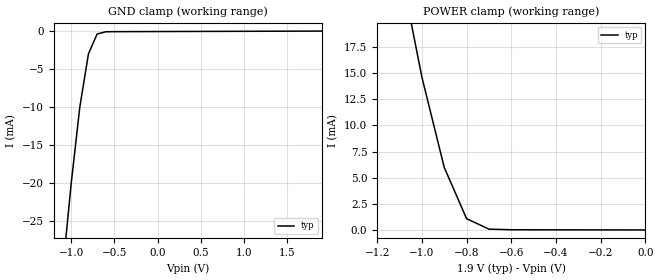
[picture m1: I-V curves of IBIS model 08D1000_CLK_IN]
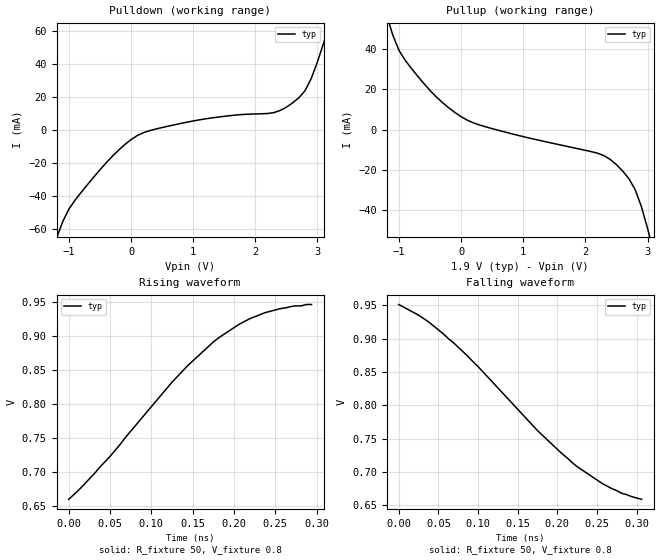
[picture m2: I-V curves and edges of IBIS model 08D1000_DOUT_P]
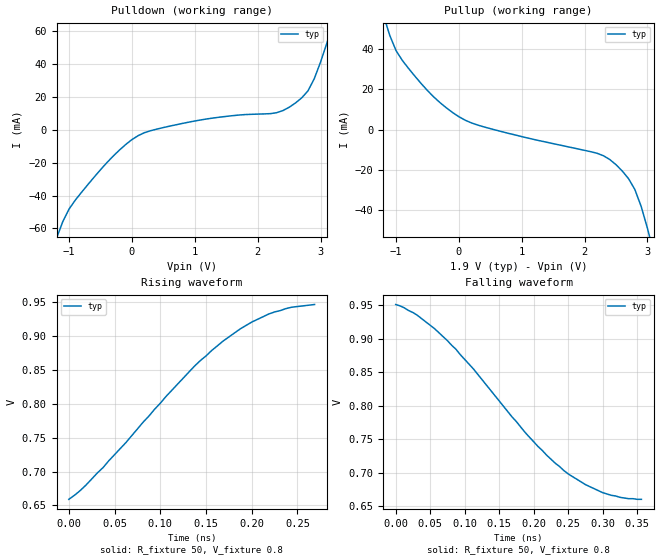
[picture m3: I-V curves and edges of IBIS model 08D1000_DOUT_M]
|   National Semiconductor Corporation
|   Data Conversion Products Group
|   IBIS Model of ADC08D1000
|   128 Pin Exposed Pad LQFP Package
[IBIS Ver]   3.2
[File name]   adc08d1000.ibs
[File Rev]   1.1
[Date]   08/11/06
[Source]   Bench Test to Ibis Conversion.
[Notes]   File created by Ian King
   Updated by Craig Klem  -  Fixed [Diff-pin] to allow
   LineSim simulations
[Disclaimer]
(C) Copyright National Semiconductor Corporation 2006
   All rights reserved
   National Semiconductor Corporation hereby grants
the user of this IBIS model a non-exclusive, nontransferable
license to use this IBIS model under the following terms.
Before using this IBIS model, the user should read this
license.  If the user does not accept these terms,  the
IBIS model should be returned to National within 30 days.
   The user is granted this license only to use the
IBIS model and is not granted rights to sell, load, rent,
lease or license the IBIS model in whole or in part, or in
modified form to anyone other than user. User may modify
the IBIS model to suit its specific applications but rights
to derivative works and such modifications shall belong to
National.
   This IBIS model is provided on an "AS IS" basis and
National makes absolutely no warranty with respect to the
information contained herein.NATIONAL DISCLAIMS AND CUSTOMER
WAIVES ALL WARRANTIES, EXPRESS OR IMPLIED, INCLUDING
WARRANTIES OF MERCHANTABILITY OR FITNESS FOR A PARTICULAR
PURPOSE. The entire risk as to quality and performance is
with the Customer. ACCORDINGLY, IN NO EVENT SHALL THE
COMPANY BE LIABLE FOR ANY DAMAGES, WHETHER IN CONTRACT OR
TORT,INCLUDING ANY LOST PROFITS OR OTHER INCIDENTAL,
CONSEQUENTIAL, EXEMPLARY, OR PUNITIVE DAMAGES ARISING OUT
OF THE USE OR APPLICATION OF THE IBIS model provided in
this package.Further, National reserves the right to make
changes without notice to any product herein to improve
reliability, function, or design. National does not convey
any license under patent rights or any other intellectual
property rights, including those of third parties.
   National is not obligated to provide maintenance or support
for the licensed IBIS model.
Contact National at ATTN:DCS APPLICATIONS/IBIS MODELS.
2900 Semiconductor Drive, M/S D3-739, Santa Clara, CA 95052-8090
[Copyright]   Copyright 2006, National Semiconductor, All Rights Reserved
[Component]   ADC08D1000
[Manufacturer]  National Semiconductor Corp
[Package]
|   typ   min   max
R_pkg   416.0m   397.0m   444.0m
L_pkg   8.66n   7.94n   10.10n
C_pkg   0.10p   0.09p   0.14p
[Pin]   signal_name   model_name   R_pin   L_pin   C_pin
1   GND   GND   426.0m   10.1n   0.14p
2   VA   POWER   431.0m   9.78n   0.12p
3   OUTV/SCLK   NC
4   OE/DDR/SDATA   NC
5   VA   POWER   444.0m   9.14n   0.10p
6   GND   GND   435.0m   8.93n   0.10p
7   VCMO   NC
8   VA   POWER   417.0m   8.52n   0.10p
9   GND   GND   408.0m   8.31n   0.10p
10   VINI-   NC   407.0m   8.23n   0.10p
11   VINI+   NC   403.0m   8.18n   0.10p
12   GND   GND   397.0m   7.94n   0.10p
13   VA   POWER   397.0m   8.04n   0.09p
14   FSR/ECE   NC
15   DCLK_RST   NC
16   VA   POWER   397.0m   7.99n   0.09p
17   VA   POWER   397.0m   7.99n   0.09p
18   CLK+   08D1000_CLK_IN   397.0m   7.99n   0.09p
19   CLK-   08D1000_CLK_IN   397.0m   7.99n   0.09p
20   VA   POWER   397.0m   8.04n   0.09p
21   GND   GND   397.0m   7.94n   0.10p
22   VINQ+   NC   403.0m   8.18n   0.10p
23   VINQ-   NC   407.0m   8.23n   0.10p
24   GND   GND   408.0m   8.31n   0.10p
25   VA   POWER   417.0m   8.52n   0.10p
26   PD   NC
27   GND   GND   435.0m   8.93n   0.10p
28   VA   POWER   444.0m   9.14n   0.10p
29   PDQ   NC
30   CAL   NC
31   VBG   NC
32   REXT   NC
33   VA   POWER   426.0m   10.1n   0.14p
34   TDIODE_P   NC
35   TDIODE_N   NC
36   DQD0+   08D1000_DOUT_P   444.0m   9.27n   0.10p
37   DQD0-   08D1000_DOUT_M   444.0m   9.14n   0.10p
38   DQD1+   08D1000_DOUT_P   435.0m   8.93n   0.10p
39   DQD1-   08D1000_DOUT_M   426.0m   8.73n   0.10p
40   VDR   POWER   417.0m   8.52n   0.10p
41   GND   GND   408.0m   8.31n   0.10p
42   DRGND   GND   407.0m   8.23n   0.10p
43   DQD2+   08D1000_DOUT_P   403.0m   8.18n   0.10p
44   DQD2-   08D1000_DOUT_M   397.0m   7.94n   0.10p
45   DQD3+   08D1000_DOUT_P   397.0m   8.04n   0.09p
46   DQD3-   08D1000_DOUT_M   397.0m   7.99n   0.09p
47   DQD4+   08D1000_DOUT_P   397.0m   7.99n   0.09p
48   DQD4-   08D1000_DOUT_M   397.0m   7.99n   0.09p
49   DQD5+   08D1000_DOUT_P   397.0m   7.99n   0.09p
50   DQD5-   08D1000_DOUT_M   397.0m   7.99n   0.09p
51   VDR   POWER   397.0m   7.99n   0.09p
52   NC   NC
53   DRGND   GND   397.0m   7.94n   0.10p
54   DQD6+   08D1000_DOUT_P   403.0m   8.18n   0.10p
55   DQD6-   08D1000_DOUT_M   407.0m   8.23n   0.10p
56   DQD7+   08D1000_DOUT_P   408.0m   8.31n   0.10p
57   DQD7-   08D1000_DOUT_M   417.0m   8.52n   0.10p
58   DQ0+   08D1000_DOUT_P   426.0m   8.73n   0.10p
59   DQ0-   08D1000_DOUT_M   435.0m   8.93n   0.10p
60   DQ1+   08D1000_DOUT_P   444.0m   9.14n   0.10p
61   DQ1-   08D1000_DOUT_M   444.0m   9.27n   0.10p
62   VDR   POWER   436.0m   9.78n   0.10p
63   NC   NC
64   DRGND   GND   426.0m   10.1n   0.14p
65   DQ2+   08D1000_DOUT_P   426.0m   10.1n   0.14p
66   DQ2-   08D1000_DOUT_M   431.0m   9.78n   0.12p
67   DQ3+   08D1000_DOUT_P   436.0m   9.42n   0.10p
68   DQ3-   08D1000_DOUT_M   444.0m   9.27n   0.10p
69   DQ4+   08D1000_DOUT_P   444.0m   9.14n   0.10p
70   DQ4-   08D1000_DOUT_M   435.0m   8.93n   0.10p
71   DQ5+   08D1000_DOUT_P   426.0m   8.73n   0.10p
72   DQ5-   08D1000_DOUT_M   417.0m   8.52n   0.10p
73   VDR   POWER   408.0m   8.31n   0.10p
74   DRGND   GND   407.0m   8.23n   0.10p
75   DQ6+   08D1000_DOUT_P   403.0m   8.18n   0.10p
76   DQ6-   08D1000_DOUT_M   397.0m   7.94n   0.10p
77   DQ7+   08D1000_DOUT_P   397.0m   7.99n   0.09p
78   DQ7-   08D1000_DOUT_M   397.0m   7.99n   0.09p
79   OR+   NC
80   OR-   NC
81   DCLK-   08D1000_DCLK_M   397.0m   7.99n   0.09p
82   DCLK+   08D1000_DCLK_P   397.0m   7.99n   0.09p
83   DI7-   08D1000_DOUT_M   397.0m   7.99n   0.09p
84   DI7+   08D1000_DOUT_P   397.0m   8.04n   0.09p
85   DI6-   08D1000_DOUT_M   397.0m   7.94n   0.10p
86   DI6+   08D1000_DOUT_P   403.0m   8.18n   0.10p
87   DRGND   GND   407.0m   8.23n   0.10p
88   VDR   POWER   408.0m   8.31n   0.10p
89   DI5-   08D1000_DOUT_M   417.0m   8.52n   0.10p
90   DI5+   08D1000_DOUT_P   426.0m   8.73n   0.10p
91   DI4-   08D1000_DOUT_M   435.0m   8.93n   0.10p
92   DI4+   08D1000_DOUT_P   444.0m   9.14n   0.10p
93   DI3-   08D1000_DOUT_M   444.0m   9.27n   0.10p
94   DI3+   08D1000_DOUT_P   436.0m   9.42n   0.10p
95   DI2-   08D1000_DOUT_M   431.0m   9.78n   0.12p
96   DI2+   08D1000_DOUT_P   426.0m   10.1n   0.14p
97   DRGND   GND   426.0m   10.1n   0.14p
98   NC   NC
99   VDR   POWER   436.0m   9.42n   0.10p
100   DI1-   08D1000_DOUT_M   444.0m   9.27n   0.10p
101   DI1+   08D1000_DOUT_P   444.0m   9.14n   0.10p
102   DI0-   08D1000_DOUT_M   435.0m   8.93n   0.10p
103   DI0+   08D1000_DOUT_P   426.0m   8.73n   0.10p
104   DID7-   08D1000_DOUT_M   417.0m   8.52n   0.10p
105   DID7+   08D1000_DOUT_P   408.0m   8.31n   0.10p
106   DID6-   08D1000_DOUT_M   407.0m   8.23n   0.10p
107   DID6+   08D1000_DOUT_P   403.0m   8.18n   0.10p
108   DRGND   GND   397.0m   7.94n   0.10p
109   NC   NC
110   VDR   POWER   397.0m   7.99n   0.09p
111   DID5-   08D1000_DOUT_M   397.0m   7.99n   0.09p
112   DID5+   08D1000_DOUT_P   397.0m   7.99n   0.09p
113   DID4-   08D1000_DOUT_M   397.0m   7.99n   0.09p
114   DID4+   08D1000_DOUT_P   397.0m   7.99n   0.09p
115   DID3-   08D1000_DOUT_M   397.0m   7.99n   0.09p
116   DID3+   08D1000_DOUT_P   397.0m   8.04n   0.09p
117   DID2-   08D1000_DOUT_M   397.0m   7.94n   0.09p
118   DID2+   08D1000_DOUT_P   403.0m   8.18n   0.10p
119   DRGND   GND   407.0m   8.23n   0.10p
120   NC   NC
121   VDR   POWER   417.0m   8.52n   0.10p
122   DID1-   08D1000_DOUT_M   426.0m   8.73n   0.10p
123   DID1+   08D1000_DOUT_P   435.0m   8.93n   0.10p
124   DID0-   08D1000_DOUT_M   444.0m   9.14n   0.10p
125   DID0+   08D1000_DOUT_P   444.0m   9.27n   0.10p
126   CALRUN   NC
127   CALDLY/DES/SCS  NC
128   VA   POWER   426.0m   10.1n   0.14p
[Diff_pin]   inv_pin   vdiff   tdelay_typ   tdelay_min   tdelay_max
| The '+' pin is Diff_pin and the '-' pin is the inv_pin
18   19   400m   NA
36   37   NA   0   0   0
38   39   NA   0   0   0
43   44   NA   0   0   0
45   46   NA   0   0   0
47   48   NA   0   0   0
49   50   NA   0   0   0
54   55   NA   0   0   0
56   57   NA   0   0   0
58   59   NA   0   0   0
60   61   NA   0   0   0
65   66   NA   0   0   0
67   68   NA   0   0   0
69   70   NA   0   0   0
71   72   NA   0   0   0
75   76   NA   0   0   0
77   78   NA   0   0   0
82   81   NA   0   0   0
84   83   NA   0   0   0
86   85   NA   0   0   0
90   89   NA   0   0   0
92   91   NA   0   0   0
94   93   NA   0   0   0
96   95   NA   0   0   0
101   100   NA   0   0   0
103   102   NA   0   0   0
105   104   NA   0   0   0
107   106   NA   0   0   0
112   111   NA   0   0   0
114   113   NA   0   0   0
116   115   NA   0   0   0
118   117   NA   0   0   0
123   122   NA   0   0   0
125   124   NA   0   0   0
| Models and submodels in the file (5): 08D1000_CLK_IN (Input), 08D1000_DOUT_P (Output), 08D1000_DOUT_M (Output), 08D1000_DCLK_P (Output), 08D1000_DCLK_M (Output)
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|   Clock Input MODEL
[Model]   08D1000_CLK_IN
Model_type Input
Vinh=0.2
Vinl=-0.2
|   TYP   MIN   MAX
C_comp   1.5p   1.5p   1.5p
[Temperature Range] 25   85   -40
[Voltage Range]   1.90   1.80   2.00
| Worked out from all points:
|   GND clamp passes 1 mA (typ) near -0.72 V on its own axis
|   POWER clamp passes 1 mA (typ) near -0.79 V on its own axis
[GND Clamp]
|V(groundclamp)   I(typ)   I(min)   I(max)
-1.9V     -557.1mA   NA         NA
-1.1V     -31.82mA   NA         NA
-1V       -20.11mA   NA         NA
-900mV    -9.993mA   NA         NA
-800mV    -2.979mA   NA         NA
-700mV    -364uA     NA         NA
-600mV    -66uA      NA         NA
-500mV    -51uA      NA         NA
1.9V      25uA       NA         NA
[POWER Clamp]
|V(table)   I(typ)   I(min)   I(max)
-1.9V     612.9mA    NA         NA
-1.1V     25.42mA    NA         NA
-1V       14.61mA    NA         NA
-900mV    5.99mA     NA         NA
-800mV    1.101mA    NA         NA
-700mV    104.3uA    NA         NA
0V        24.8uA     NA         NA
|   Driver Output MODELs
[Model]   08D1000_DOUT_P
Model_type Output
Polarity Non-Inverting
Vref=0.80
Vmeas=0.80
Rref=50
Cref=5p
|   TYP   MIN   MAX
C_comp   1.5p   1.5p   1.5p
[Temperature Range] 25   85   -40
[Voltage Range]   1.90   1.80   2.00
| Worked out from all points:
|   slope of the pulldown table from 0 to 0.285 V, typ, clamps not added: 54.2 ohm
|   slope of the pullup table from 0 to 0.285 V, typ, clamps not added: 71.2 ohm
|   falling waveform, R_fixture 50, V_fixture 0.8: 20-80 % time 146ps typ, NA min, NA max; typ from 0.951 V to 0.659 V
|   rising waveform, R_fixture 50, V_fixture 0.8: 20-80 % time 128ps typ, NA min, NA max; typ from 0.66 V to 0.946 V
[Pullup]
|Vtable   I(typ)   I(min)   I(max)
-1.9V     504.4mA    NA         NA
-1.2V     56.99mA    NA         NA
-1V       39.3mA     NA         NA
-700mV    26.59mA    NA         NA
0V        6.476mA    NA         NA
500mV     541uA      NA         NA
2.3V      -12.87mA   NA         NA
2.7V      -24.26mA   NA         NA
2.8V      -29.63mA   NA         NA
3V        -48.87mA   NA         NA
3.1V      -61.09mA   NA         NA
3.8V      -629.5mA   NA         NA
[Pulldown]
|V(pulldown)   I(typ)   I(min)   I(max)
-1.9V     -631mA     NA         NA
-1.2V     -65.78mA   NA         NA
-1V       -48.04mA   NA         NA
-500mV    -24.23mA   NA         NA
-100mV    -8.945mA   NA         NA
200mV     -1.752mA   NA         NA
2.3V      10.4mA     NA         NA
2.5V      13.68mA    NA         NA
2.8V      23.66mA    NA         NA
2.9V      31.05mA    NA         NA
3.2V      64.91mA    NA         NA
3.8V      503.6mA    NA         NA
[Ramp]
|   TYP   MIN   MAX
dV/dt_r   164mv/.122ns   NA   NA
dV/dt_f   164mv/.136ns   NA   NA
R_load=50
[Falling Waveform]
R_fixture=50
V_fixture=0.8
| 100 Ohms Across Outputs DOUTP and DOUTM
|Time   V(typ)   V(min)   V(max)
0s        951mV      NA         NA
37.5ps    925mV      NA         NA
68.8ps    894mV      NA         NA
100ps     858mV      NA         NA
175ps     762mV      NA         NA
225ps     708mV      NA         NA
256.3ps   683mV      NA         NA
268.8ps   675mV      NA         NA
281.3ps   668mV      NA         NA
306.3ps   659mV      NA         NA
[Rising Waveform]
R_fixture=50
V_fixture=0.8
|Time   V(typ)   V(min)   V(max)
0s        660mV      NA         NA
12.5ps    674mV      NA         NA
50ps      723mV      NA         NA
125ps     832mV      NA         NA
143.8ps   856mV      NA         NA
175ps     891mV      NA         NA
206.3ps   917mV      NA         NA
237.5ps   934mV      NA         NA
268.8ps   943mV      NA         NA
293.8ps   946mV      NA         NA
[Model]   08D1000_DOUT_M
Model_type Output
Polarity Inverting
Vref=0.80
Vmeas=0.80
Rref=50   | 100 Ohms Across Outputs OUTP and OUTM
Cref=5p
|   TYP   MIN   MAX
C_comp   1.5p   1.5p   1.5p
[Temperature Range] 25   85   -40
[Voltage Range]   1.90   1.80   2.00
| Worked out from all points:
|   slope of the pulldown table from 0 to 0.285 V, typ, clamps not added: 54.4 ohm
|   slope of the pullup table from 0 to 0.285 V, typ, clamps not added: 71.2 ohm
|   falling waveform, R_fixture 50, V_fixture 0.8: 20-80 % time 148ps typ, NA min, NA max; typ from 0.951 V to 0.66 V
|   rising waveform, R_fixture 50, V_fixture 0.8: 20-80 % time 121ps typ, NA min, NA max; typ from 0.659 V to 0.947 V
[Pullup]
|Vtable   I(typ)   I(min)   I(max)
-1.9V     504.2mA    NA         NA
-1.2V     57.06mA    NA         NA
-1V       39.39mA    NA         NA
-700mV    26.66mA    NA         NA
0V        6.492mA    NA         NA
500mV     553uA      NA         NA
2.3V      -12.92mA   NA         NA
2.7V      -24.35mA   NA         NA
2.8V      -29.75mA   NA         NA
3V        -49.01mA   NA         NA
3.1V      -61.26mA   NA         NA
3.8V      -634.3mA   NA         NA
[Pulldown]
|V(pulldown)   I(typ)   I(min)   I(max)
-1.9V     -635.7mA   NA         NA
-1.2V     -65.92mA   NA         NA
-1V       -48.17mA   NA         NA
-500mV    -24.3mA    NA         NA
-100mV    -8.977mA   NA         NA
200mV     -1.775mA   NA         NA
2.3V      10.34mA    NA         NA
2.5V      13.65mA    NA         NA
2.8V      23.66mA    NA         NA
2.9V      31.08mA    NA         NA
3.2V      64.97mA    NA         NA
3.8V      503.7mA    NA         NA
[Ramp]
|   TYP   MIN   MAX
dV/dt_r   164mv/.118ns   NA   NA
dV/dt_f   164mv/.138ns   NA   NA
R_load=50
[Falling Waveform]
R_fixture=50
V_fixture=0.8
|Time   V(typ)   V(min)   V(max)
0s        951mV      NA         NA
31.2ps    935mV      NA         NA
75ps      897mV      NA         NA
112.5ps   855mV      NA         NA
187.5ps   760mV      NA         NA
243.7ps   703mV      NA         NA
275ps     682mV      NA         NA
300ps     670mV      NA         NA
325ps     663mV      NA         NA
356.2ps   660mV      NA         NA
[Rising Waveform]
R_fixture=50
V_fixture=0.8
|Time   V(typ)   V(min)   V(max)
0s        659mV      NA         NA
12.5ps    672mV      NA         NA
37.5ps    706mV      NA         NA
106.2ps   811mV      NA         NA
137.5ps   856mV      NA         NA
168.7ps   893mV      NA         NA
193.7ps   916mV      NA         NA
218.7ps   933mV      NA         NA
243.7ps   943mV      NA         NA
268.7ps   947mV      NA         NA
